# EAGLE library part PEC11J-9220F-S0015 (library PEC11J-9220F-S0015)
12 mm SMD Long Life Encoder Source: Datasheet
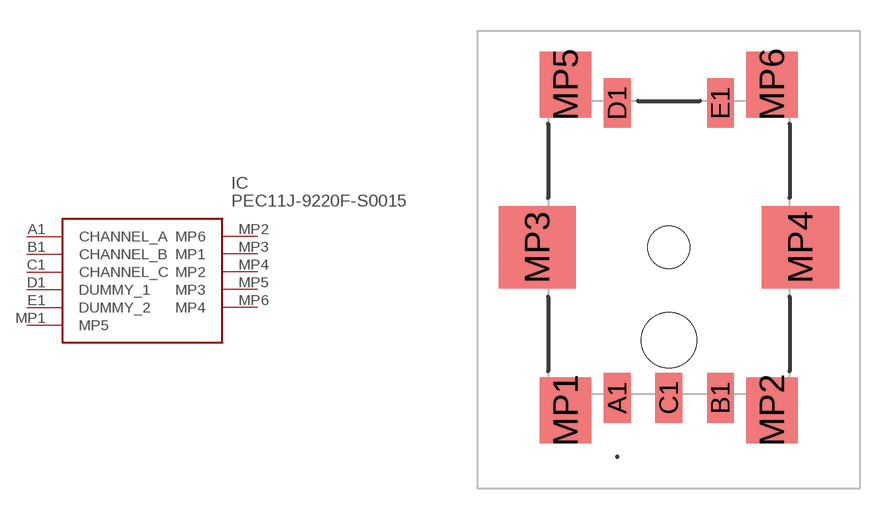
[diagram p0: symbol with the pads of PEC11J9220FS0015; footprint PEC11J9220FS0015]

Designator prefix IC

## PEC11J-9220F-S0015 (Description: 12 mm SMD Long Life Encoder; Height: 25mm; Manufacturer_Name: Bourns; Manufacturer_Part_Number: PEC11J-9220F-S0015; Mouser_Part_Number: 652-PEC11J9220FS0015; Mouser_Price-Stock: https://www.mouser.co.uk/ProductDetail/Bourns/PEC11J-9220F-S0015?qs=11PymoJGorKK%252Ba0mQ8KVhA%3D%3D)  [PEC11J9220FS0015]
A1  CHANNEL_A
B1  CHANNEL_B
C1  CHANNEL_C
D1  DUMMY_1
E1  DUMMY_2
MP1  MP5
MP2  MP6
MP3  MP1
MP4  MP2
MP5  MP3
MP6  MP4

## Footprint PEC11J9220FS0015 (pad centres in mm)
PEC11J-9220F-S0015-1
smd 1.3 x 2.4: A1 -2.5,-7.3; B1 2.5,-7.3; C1 0,-7.3; D1 -2.5,7; E1 2.5,7
smd 2.5 x 3.2: MP1 -5,-7.9; MP2 5,-7.9; MP5 -5,7.9; MP6 5,7.9
smd 3.75 x 4: MP3 -6.375,0; MP4 6.375,0
hole 2.69 at 0,-4.5
hole 2.05 at 0,0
